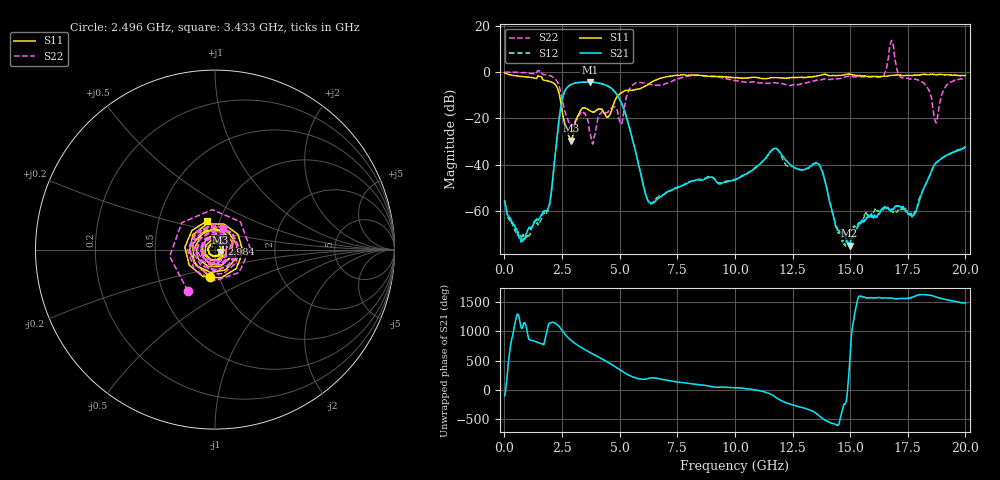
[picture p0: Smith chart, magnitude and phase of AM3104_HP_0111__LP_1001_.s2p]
!Created with skrf (http://scikit-rf.org).
# Hz S RI R 50.0
!freq ReS11 ImS11 ReS21 ImS21 ReS12 ImS12 ReS22 ImS22
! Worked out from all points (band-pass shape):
!   1601 points, 10 MHz to 20 GHz, reference 50 ohm
!   highest |S21| = -4.23 dB at 3.708 GHz (marker M1); lowest = -75.0 dB at 14.98 GHz (marker M2)
!   |S21| within 3 dB of the highest: 2.678 GHz to 4.668 GHz (1.99 GHz wide, 54.2 % of centre)
!   lowest |S11| = -29.6 dB at 2.884 GHz (marker M3), VSWR 1.07, Z = 53.1 - j1.37 ohm
!   |S11| at or under -10 dB: 2.39 GHz to 4.943 GHz (2.553 GHz wide, 69.6 % of centre)
!   |S22| runs from -31.1 to 13.7 dB; largest |S21 - S12| = 0.048
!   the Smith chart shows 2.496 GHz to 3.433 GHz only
!   S11 on the Smith chart (normalised r, x): 2.496 GHz: 0.91, -0.28; 2.984 GHz: 1.08, +0.06; 3.433 GHz: 0.87, +0.29
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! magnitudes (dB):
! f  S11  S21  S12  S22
! 10 MHz  -0.4  -55.6  -55.9  0.0
! 759.6 MHz  -1.9  -72.6  -71.8  -0.3
! 1.859 GHz  -3.8  -59.5  -59.9  -1.3
! 2.496 GHz  -16.3  -12.5  -12.5  -11.2
! 2.884 GHz  -29.6  -5.4  -5.5  -23.6
! 2.984 GHz  -26.4  -5.0  -5.0  -23.0
! 3.346 GHz  -16.1  -4.4  -4.5  -17.1
! 3.433 GHz  -15.6  -4.3  -4.3  -17.6
! 3.708 GHz  -16.6  -4.2  -4.3  -26.1
! 4.933 GHz  -10.1  -10.5  -10.6  -18.4
! 6.182 GHz  -5.7  -54.5  -54.1  -5.1
! 6.682 GHz  -3.0  -54.3  -53.9  -5.7
! 10.01 GHz  -2.5  -46.5  -46.6  -3.7
! 11.72 GHz  -2.4  -33.0  -33.0  -4.6
! 13.34 GHz  -2.1  -40.3  -40.2  -4.0
! 13.75 GHz  -1.3  -42.0  -41.7  -3.3
! 14.7 GHz  -1.3  -69.9  -73.3  -2.4
! 14.98 GHz  -0.9  -75.0  -69.3  -1.7
! 16.68 GHz  -1.6  -59.1  -59.2  7.3
! 17.76 GHz  -1.3  -61.8  -61.4  -3.1
! 18.71 GHz  -1.2  -39.2  -39.4  -21.7
! 20 GHz  -1.4  -32.6  -32.2  -2.6
